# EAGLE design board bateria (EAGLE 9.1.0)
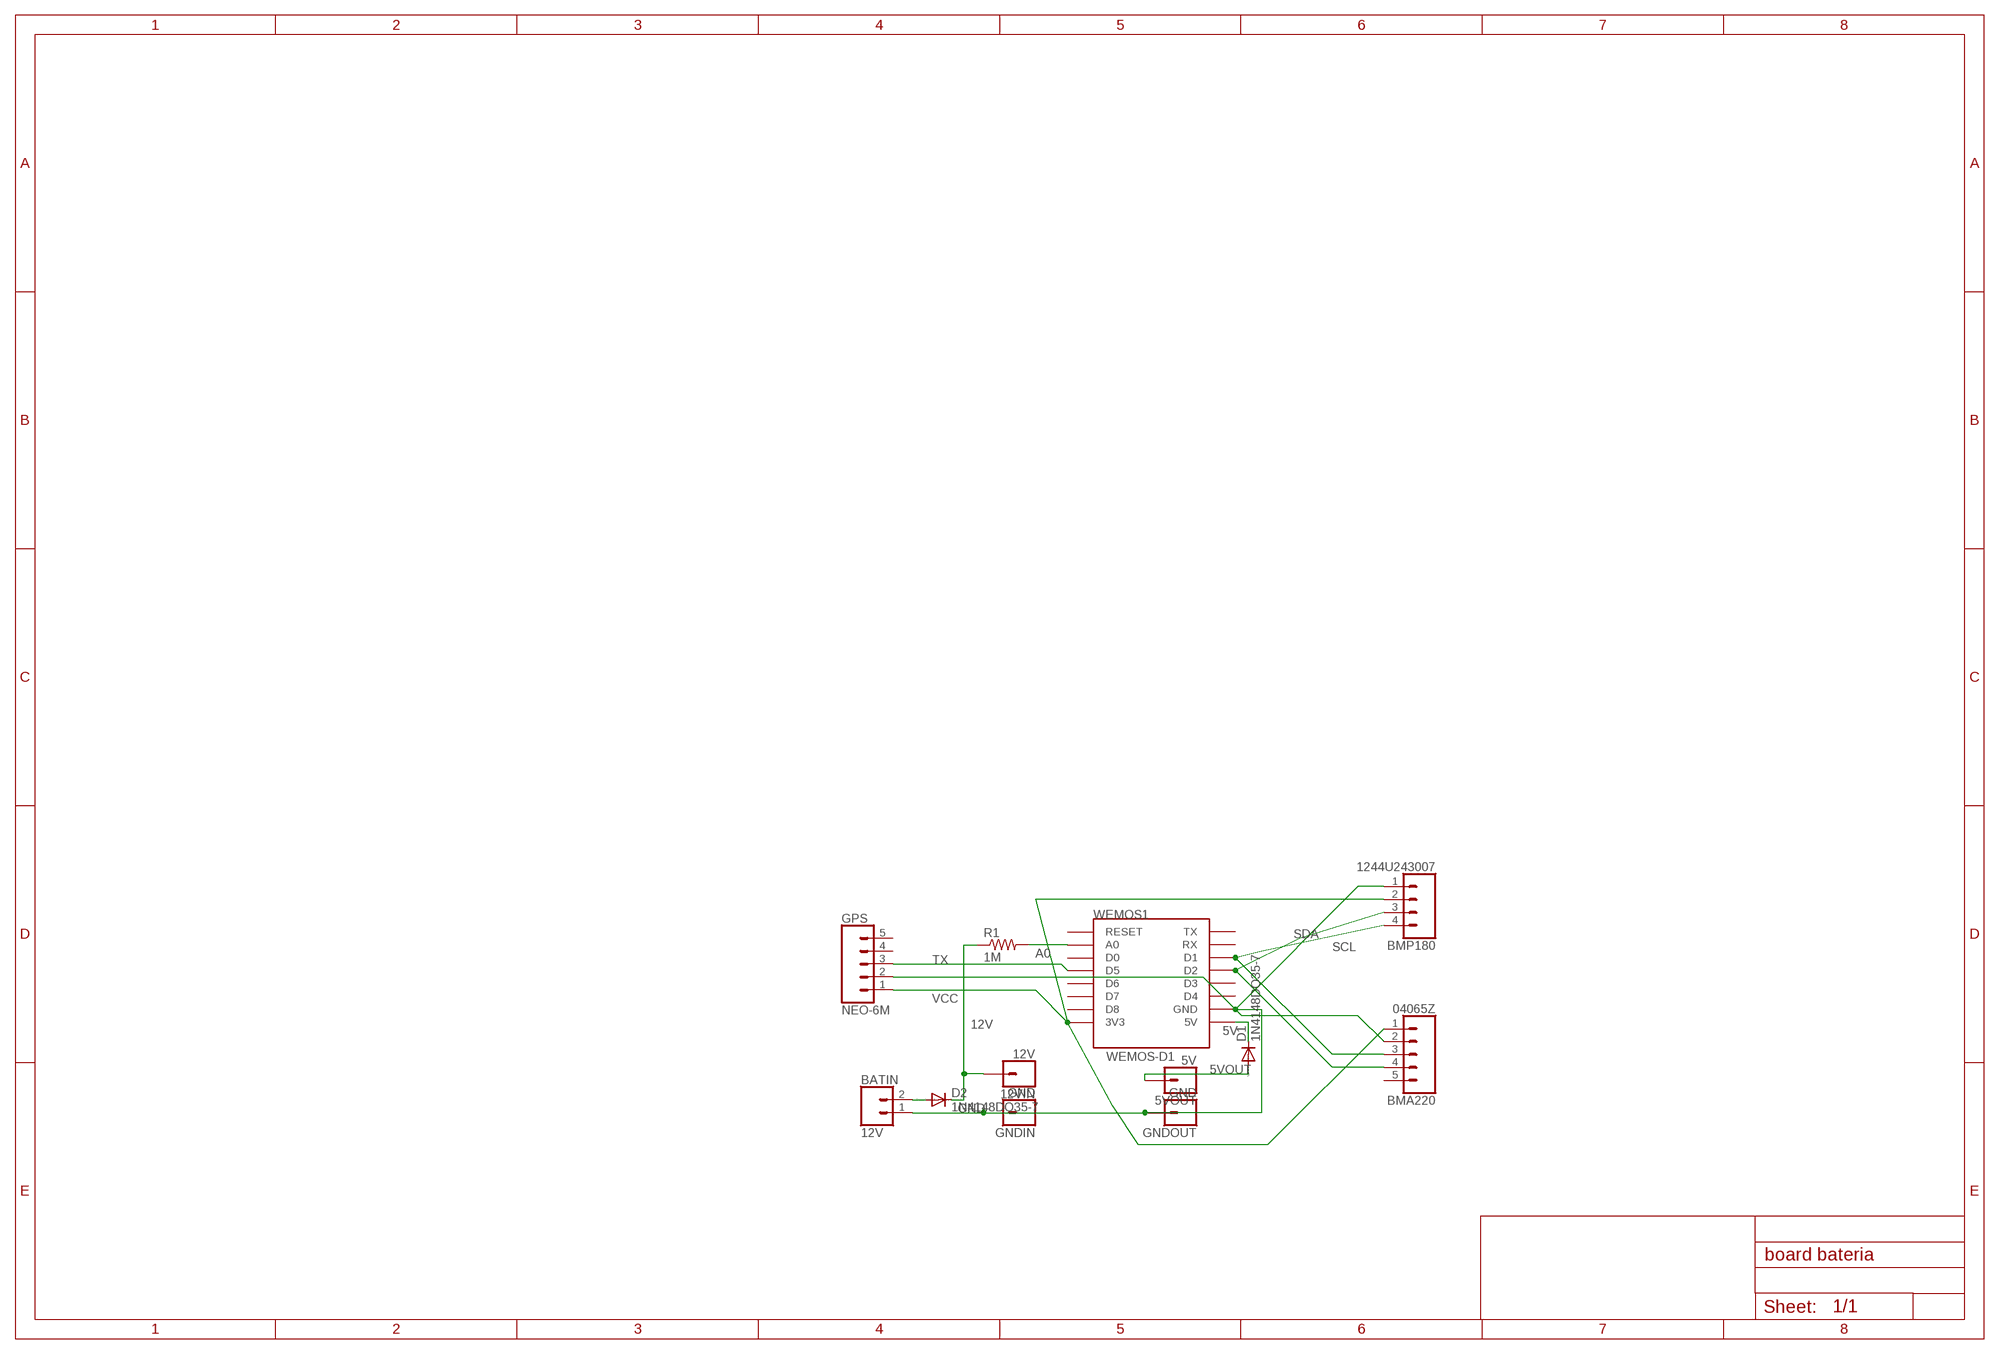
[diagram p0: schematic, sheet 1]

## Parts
5VOUT  5V  CONN_01  [1X01]
12VIN  12V  CONN_01  [1X01]
BATIN  12V  CONN_02  [1X02]
BMA220  04065Z  CONN_05  [1X05]
BMP180  1244U243007  CONN_04  [1X04]
D1  1N4148DO35-7  [DO35-7]
D2  1N4148DO35-7  [DO35-7]
GNDIN  GND  CONN_01  [1X01]
GNDOUT  GND  CONN_01  [1X01]
GPS  NEO-6M  CONN_05  [1X05]
R1  1M  R-US_R0805  [R0805]
WEMOS1  WEMOS-D1  WEMOS-D1-MINI  [WEMOS-D1-MINI]

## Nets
5V: D1.C WEMOS1.5V
5VOUT: 5VOUT.1 D1.A
12V: 12VIN.1 D2.C R1.1
A0: R1.2 WEMOS1.A0
GND: BATIN.1 BMA220.2 BMP180.1 GNDIN.1 GNDOUT.1 GPS.2 WEMOS1.GND
N$2: BATIN.2 D2.A
SCL: BMA220.3 BMP180.4 WEMOS1.D1
SDA: BMA220.4 BMP180.3 WEMOS1.D2
TX: GPS.3 WEMOS1.D5
VCC: BMA220.1 BMP180.2 GPS.1 WEMOS1.3V3
Unconnected: BMA220.5 GPS.4 GPS.5 WEMOS1.D0 WEMOS1.D3 WEMOS1.D4 WEMOS1.D6 WEMOS1.D7 WEMOS1.D8 WEMOS1.RESET WEMOS1.RX WEMOS1.TX

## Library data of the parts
5VOUT 12VIN GNDIN GNDOUT = SparkFun-Connectors:CONN_01: Single connection point. Often used as Generic Header-pin footprint for 0.1 inch spaced/style header connections
BATIN = SparkFun-Connectors:CONN_02: Multi connection point. Often used as Generic Header-pin footprint for 0.1 inch spaced/style header connections
BMA220 GPS = SparkFun-Connectors:CONN_05: Multi connection point. Often used as Generic Header-pin footprint for 0.1 inch spaced/style header connections On any of the 0.1 inch spaced packages, you can populate with these: Break Away Headers - Straight (PRT-00116) Break Away Male Headers - Right Angle (PRT-00553) Female Headers (PRT-00115)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
BMP180 = SparkFun-Connectors:CONN_04: Multi connection point. Often used as Generic Header-pin footprint for 0.1 inch spaced/style header connections On any of the 0.1 inch spaced packages, you can populate with these: Break Away Headers - Straight (PRT-00116) Break Away Male Headers - Right Angle (PRT-00553) Female Headers (PRT-00115)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; PROD_ID: CONN-09696
D1 D2 = diode:1N4148: DIODE
R1 = resistor:R-US_: RESISTOR, American symbol
WEMOS1 = esp8266modules:WEMOS-D1-MINI: WeMos.cc D1 mini ESP8266 module

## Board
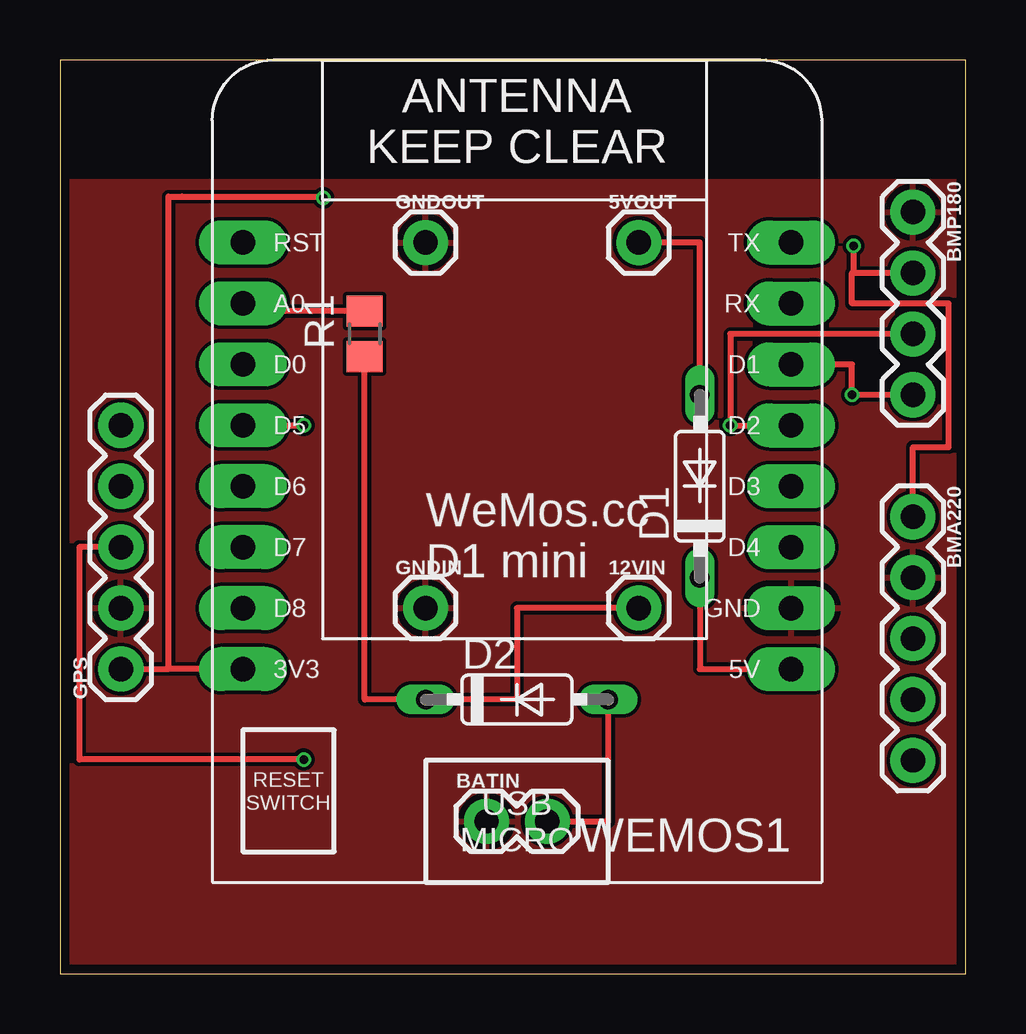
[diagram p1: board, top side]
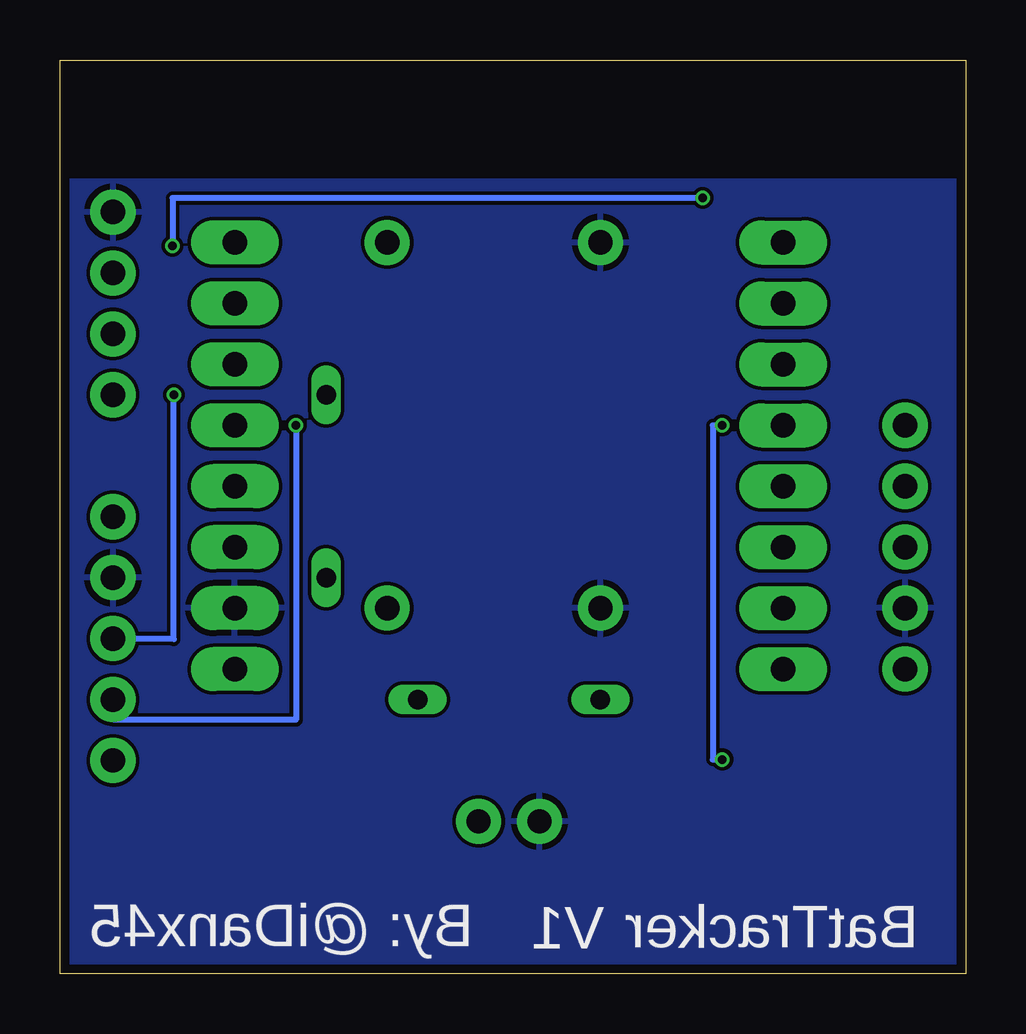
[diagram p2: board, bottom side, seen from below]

Size 37.77 x 38.09 mm. Coordinates in mm from the lower left corner, seen from the top.
Outline: 0,0 37.77,0 37.77,38.09 0,38.09 0,0
Copper layers (1*16): Top 0.035559375mm / dielectric 1.6mm / Bottom 0.035559375mm
Design rules "oshpark-2layer": minimum track width 6mil, minimum drill 10mil, track to track 6mil, track to pad 6mil, pad to pad 6mil, via to via 6mil, smd to smd 6mil, copper to edge 15mil, drill to drill 6mil, minimum pad ring 5mil, minimum via ring 5mil, stop-mask expansion 2.5mil, vias tented up to drill 0mil, thermal gap 10mil

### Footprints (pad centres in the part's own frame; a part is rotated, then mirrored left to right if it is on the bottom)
1X01 = drill 1.016 pad 1.88: 1 0,0
1X02 = drill 1.016 pad 1.88: 1 0,0; 2 2.54,0
1X05 = drill 1.016 pad 1.88: 1 0,0; 2 2.54,0; 3 5.08,0; 4 7.62,0; 5 10.16,0
1X04 = drill 1.016 pad 1.88: 1 0,0; 2 2.54,0; 3 5.08,0; 4 7.62,0
DO35-7 = drill 0.813 long: A 3.81,0; C -3.81,0
R0805 = smd 1.3 x 1.5: 1 -0.95,0; 2 0.95,0
WEMOS-D1-MINI = drill 1.016 pad 1.829 long: 3V3 -10.16,-10.16; 5V 12.7,-10.16; A0 -10.16,5.08; D0 -10.16,2.54; D1 12.7,2.54; D2 12.7,0; D3 12.7,-2.54; D4 12.7,-5.08; D5 -10.16,0; D6 -10.16,-2.54; D7 -10.16,-5.08; D8 -10.16,-7.62; GND 12.7,-7.62; RESET -10.16,7.62; RX 12.7,5.08; TX 12.7,7.62

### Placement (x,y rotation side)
5VOUT  24.13,30.48 0 top
12VIN  24.13,15.24 0 top
BATIN  17.78,6.35 0 top
BMA220  35.56,19.05 270 top
BMP180  35.56,31.75 270 top
D1  26.67,20.32 90 top
D2  19.05,11.43 0 top
GNDIN  15.24,15.24 0 top
GNDOUT  15.24,30.48 0 top
GPS  2.54,12.7 90 top
R1  12.7,26.67 90 top
WEMOS1  17.78,22.86 0 top

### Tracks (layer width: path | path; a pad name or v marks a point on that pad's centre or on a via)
5V
  Top 0.254: D1.C 26.67,12.7 WEMOS1.5V
5VOUT
  Top 0.254: D1.A 26.67,30.48 5VOUT.1
12V
  Top 0.254: R1.1 12.7,11.43 D2.C 19.05,11.43 19.05,15.24 12VIN.1
A0
  Top 0.254: R1.2 7.62,27.62 WEMOS1.A0
GND
  pour Top: 0,33.02 38.1,33.02 38.1,0 0,0
  pour Bottom: 0,33.02 38.1,33.02 38.1,0 0,0
N$2
  Top 0.254: BATIN.2 22.86,6.35 D2.A
SCL  (via drill 0.35)
  Top 0.254: BMP180.4 v33.02,24.13 33.02,25.4 WEMOS1.D1
  Bottom 0.254: BMA220.3 33.06,13.97 33.03,13.94 v33.03,24.12 v33.02,24.13
SDA  (via drill 0.35)
  Top 0.254: BMP180.3 27.94,26.67 v27.94,22.86 WEMOS1.D2
  Bottom 0.254: 35.56,10.62 35.53,10.59 | v27.94,22.86 27.96,22.84 27.98,22.84 27.93,22.79 27.93,10.59 35.53,10.59 | BMA220.4 35.56,10.62 | 35.53,10.59 35.56,10.62
TX  (via drill 0.35)
  Top 0.254: v10.16,8.93 0.81,8.93 0.81,17.78 GPS.3 | WEMOS1.D5 9.68,22.86 9.93,22.86 v10.16,22.86 | v10.16,22.86
  Bottom 0.254: v10.16,22.86 10.56,22.86 10.56,8.93 v10.16,8.93
VCC  (via drill 0.35)
  Top 0.254: BMP180.2 33.02,29.21 | BMA220.1 35.56,21.95 37.04,21.95 37.04,27.94 33.02,27.94 33.02,29.21 | 5.08,32.4 | 5.08,32.4 | v10.98,32.34 10.92,32.4 5.08,32.4 | v33.08,30.34 33.08,29.27 33.02,29.21 | 5.08,32.4 4.53,32.4 4.53,12.7 | GPS.1 4.53,12.7 | WEMOS1.3V3 4.53,12.7
  Bottom 0.254: v10.98,32.34 33.08,32.34 v33.08,30.34

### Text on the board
_bsilk: BatTracker | V1 | By: @iDanx45

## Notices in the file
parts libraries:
SparkFun-Connectors: Licensing: Creative Commons ShareAlike 4.0 International - https://creativecommons.org/licenses/by-sa/4.0
